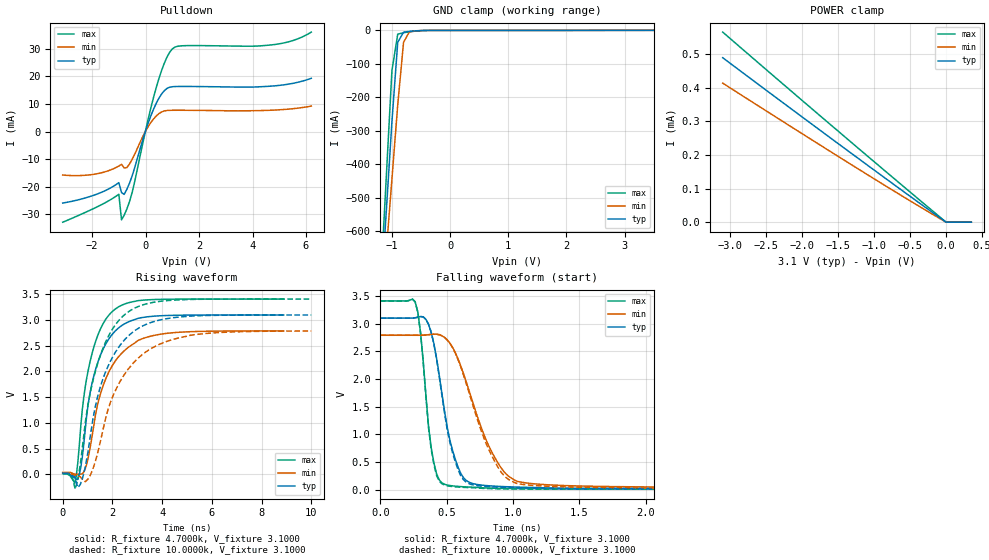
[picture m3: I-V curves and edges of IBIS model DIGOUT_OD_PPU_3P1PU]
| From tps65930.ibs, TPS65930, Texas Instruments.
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|   Model DIGOUT_OD_PPU_3P1PU
[Model]   DIGOUT_OD_PPU_3P1PU
Model_type   I/O_open_drain
Polarity   Non-Inverting
Enable   Active-Low
Vmeas =   1.6500V
Cref =  30.0000pF
Rref = 100.0000M
Vref =  0.000V
C_comp   1.0815pF   1.5672pF   1.3441pF
[Temperature Range]   25.0000   0.1250k   -40.0000
[Pullup Reference]   3.1000V   2.7900V   3.4100V
[Pulldown Reference]   0.000V   0.000V   0.000V
[POWER Clamp Reference]   3.1000V   2.7900V   3.4100V
[GND Clamp Reference]   0.000V   0.000V   0.000V
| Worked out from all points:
|   slope of the pulldown table from 0 to 0.465 V, typ, clamps not added: 41.5 ohm
|   GND clamp passes 1 mA (typ) near -0.53 V on its own axis
|   rising waveform, R_fixture 4.7000k, V_fixture 3.1000: 20-80 % time 818ps typ, 1.04ns min, 745ps max; typ from 0.022 V to 3.1 V
|   rising waveform, R_fixture 10.0000k, V_fixture 3.1000: 20-80 % time 1.19ns typ, 1.5ns min, 1.05ns max; typ from 0.01 V to 3.1 V
|   falling waveform, R_fixture 4.7000k, V_fixture 3.1000: 20-80 % time 138ps typ, 256ps min, 80.8ps max; typ from 3.1 V to 0.022 V
|   falling waveform, R_fixture 10.0000k, V_fixture 3.1000: 20-80 % time 134ps typ, 245ps min, 79.3ps max; typ from 3.1 V to 0.01 V
[Pulldown]
| voltage   I(typ)   I(min)   I(max)
-3.1V     -25.86mA   -15.72mA   -32.81mA
-1.9V     -22.92mA   -15.41mA   -27.66mA
-1V       -18.48mA   -12.46mA   -22.71mA
-900mV    -22.07mA   -11.87mA   -31.95mA
-800mV    -22.74mA   -13.16mA   -30.26mA
-500mV    -15.99mA   -10.03mA   -21.96mA
0V        267.7uA    164.1uA    390.9uA
400mV     10.28mA    5.665mA    15.99mA
700mV     14.82mA    7.491mA    24.76mA
1V        16.25mA    7.725mA    29.96mA
4.8V      16.55mA    7.792mA    31.51mA
6.2V      19.31mA    9.243mA    36.04mA
[GND_clamp]
| voltage   I(typ)   I(min)   I(max)
-3.1V     -6.084A    -5.118A    -7.02A
-1.2V     -826.4mA   -889.9mA   -777.5mA
-1.1V     -549.9mA   -667.4mA   -449.1mA
-1V       -273.4mA   -445mA     -120.7mA
-900mV    -35.57mA   -222.7mA   -11.37mA
-800mV    -5.544mA   -35.82mA   -7.069mA
-700mV    -3.081mA   -4.465mA   -4.508mA
-600mV    -1.671mA   -1.536mA   -2.434mA
-300mV    -272.6uA   -179uA     -394.9uA
3.5V      0A         0A         0A
[POWER_clamp]
| voltage   I(typ)   I(min)   I(max)
-3.1V     489.9uA    414.2uA    566.3uA
-1.2V     187uA      156uA      216.8uA
0V        0A         3.198nA    35.55pA
350mV     0A         0A         0A
[Ramp]
| variable   typ   min   max
dV/dt_r   8.0240m/0.1281n   4.9229m/0.5128n   11.6942m/0.5686n
dV/dt_f   0.4848/0.2715n   0.2278/0.3960n   0.9267/0.2170n
R_load = 50.0000
[Rising Waveform]
R_fixture = 4.7000k
V_fixture = 3.1000
V_fixture_min = 2.7900
V_fixture_max = 3.4100
| time   V(typ)   V(min)   V(max)
0s        22.04mV    33.68mV    16.54mV
484.8ps   -42.38mV   2.694mV    -175.2mV
606.1ps   -101.4mV   -2.219mV   215.8mV
727.3ps   134.5mV    -117.9uV   938.5mV
909.1ps   880.7mV    108.1mV    1.708V
1.091ns   1.557V     482.2mV    2.171V
1.515ns   2.314V     1.559V     2.825V
2.061ns   2.761V     2.164V     3.195V
3.758ns   3.08V      2.711V     3.402V
8.889ns   3.1V       2.79V      3.41V
[Rising Waveform]
R_fixture = 10.0000k
V_fixture = 3.1000
V_fixture_min = 2.7900
V_fixture_max = 3.4100
| time   V(typ)   V(min)   V(max)
0s        10.35mV    15.78mV    7.777mV
505.1ps   -90.68mV   -20.79mV   -291.5mV
707.1ps   -201.7mV   -49.4mV    188.1mV
1.01ns    417.3mV    -99.05mV   1.341V
1.414ns   1.529V     428.4mV    2.169V
1.919ns   2.201V     1.398V     2.759V
2.626ns   2.686V     2.04V      3.156V
3.636ns   2.967V     2.468V     3.345V
5.152ns   3.079V     2.706V     3.403V
10ns      3.1V       2.789V     3.41V
[Falling Waveform]
R_fixture = 4.7000k
V_fixture = 3.1000
V_fixture_min = 2.7900
V_fixture_max = 3.4100
| time   V(typ)   V(min)   V(max)
0s        3.1V       2.79V      3.41V
262.6ps   3.105V     2.79V      3.396V
303ps     3.128V     2.79V      2.847V
363.6ps   2.989V     2.8V       1.148V
404ps     2.638V     2.809V     484.6mV
525.3ps   884.8mV    2.644V     73.2mV
646.5ps   166.8mV    1.956V     48.47mV
868.7ps   61.2mV     555.9mV    23.92mV
1.111ns   40.7mV     116.9mV    17.88mV
10ns      22.04mV    33.68mV    16.54mV
[Falling Waveform]
R_fixture = 10.0000k
V_fixture = 3.1000
V_fixture_min = 2.7900
V_fixture_max = 3.4100
| time   V(typ)   V(min)   V(max)
0s        3.1V       2.79V      3.41V
262.6ps   3.105V     2.79V      3.396V
303ps     3.129V     2.79V      2.841V
363.6ps   2.988V     2.8V       1.117V
404ps     2.631V     2.81V      452.7mV
525.3ps   842.7mV    2.642V     60.34mV
626.3ps   179.6mV    2.077V     40.42mV
848.5ps   48mV       572.1mV    16.03mV
1.071ns   29.67mV    94.32mV    9.38mV
9.091ns   10.35mV    15.78mV    7.777mV
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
